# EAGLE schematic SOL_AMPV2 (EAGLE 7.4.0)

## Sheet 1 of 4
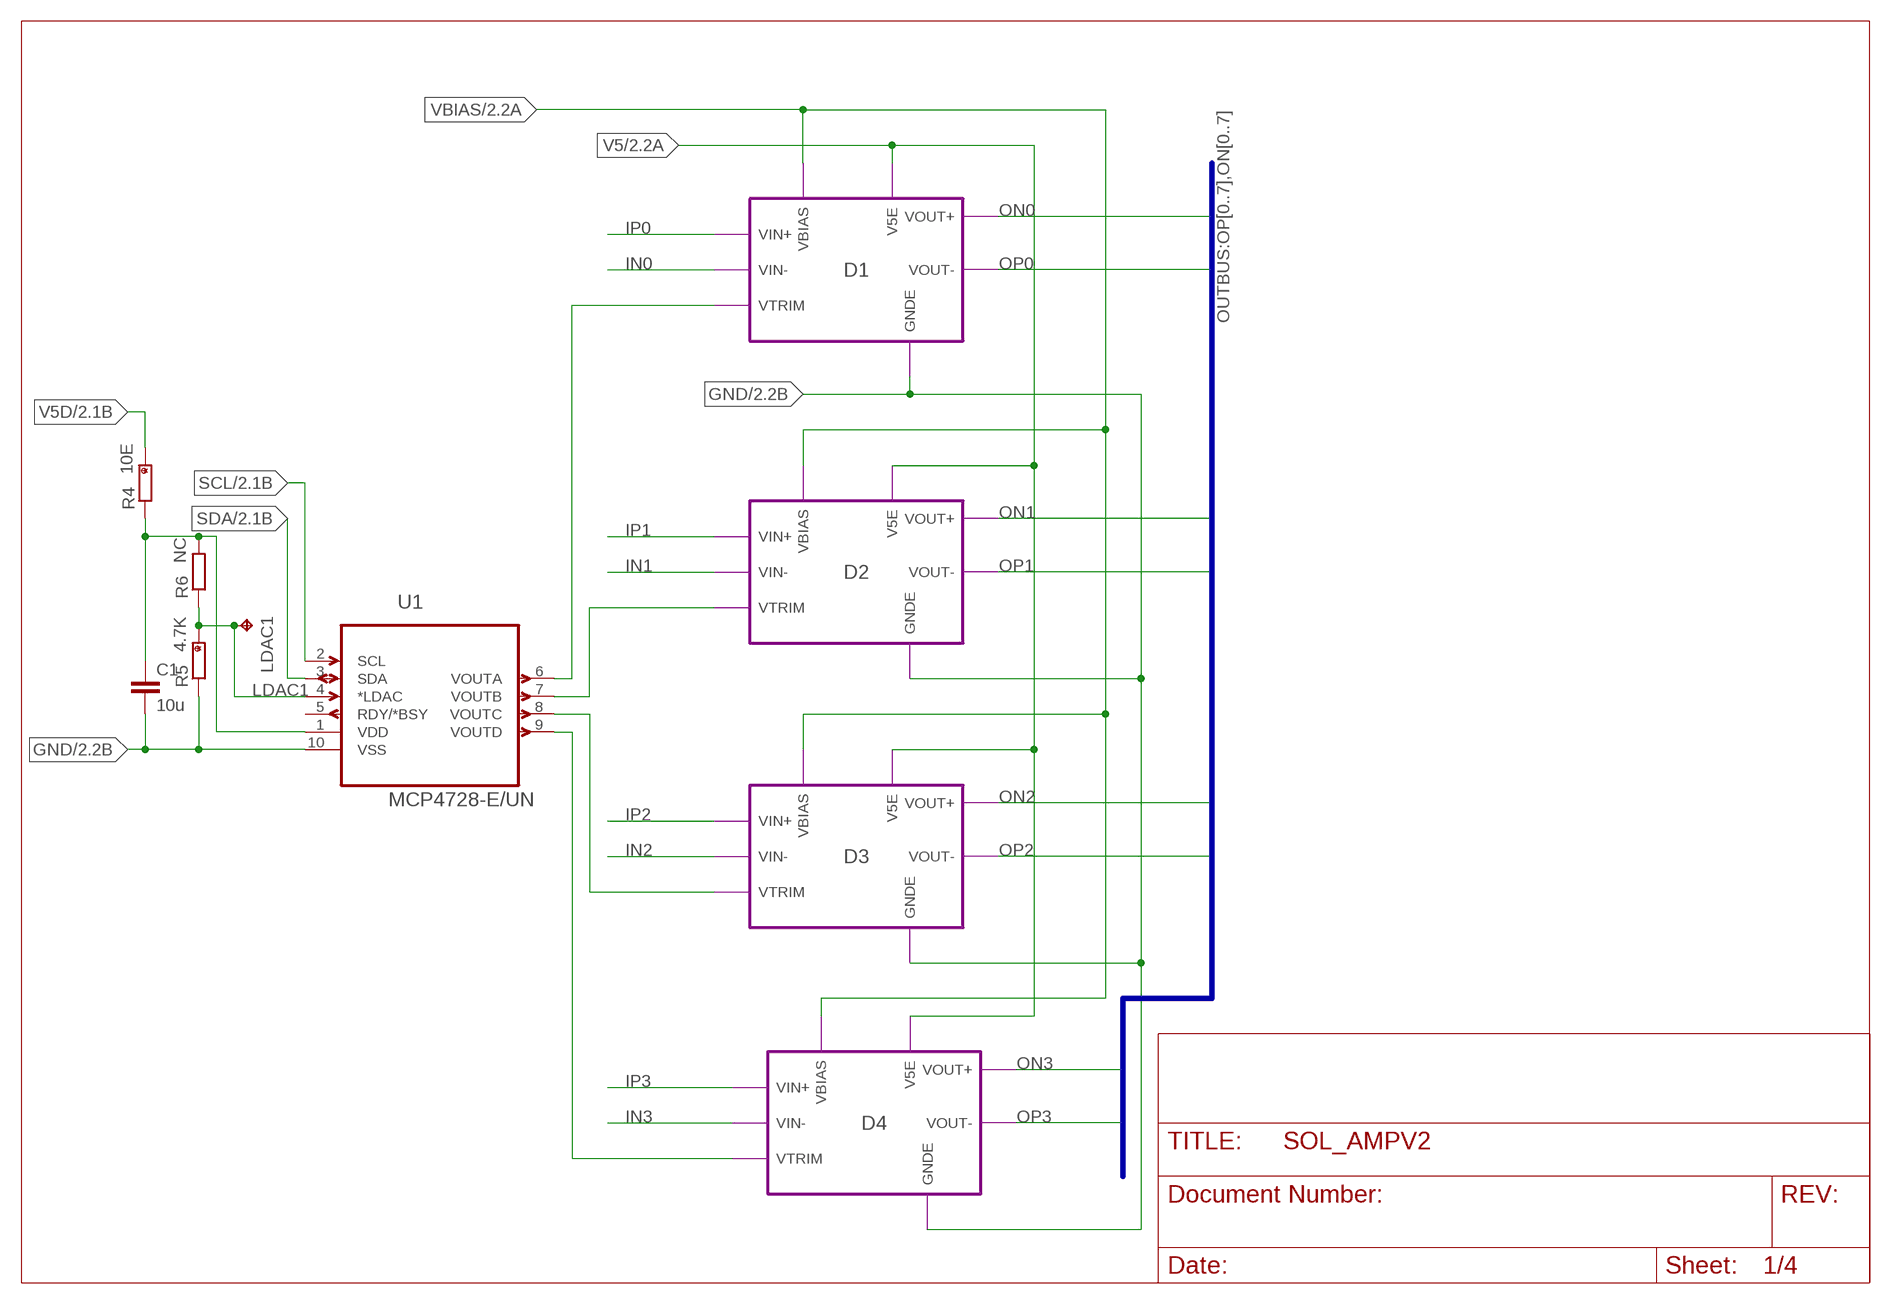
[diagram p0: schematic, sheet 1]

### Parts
C1  10u  C-EUC0805  [C0805]
LDAC1  UA_TPPAD1-13  [UA_P1-13]
R4  10E  R_HAND  [R0805H]
R5  4.7K  R_HAND  [R0805H]
R6  NC  R-EU_R0402  [R0402]
U1  MCP4728-E/UN  [SOP50P490X110-10N]

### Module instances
D2 = DIFFAMP
D1 = DIFFAMP
D3 = DIFFAMP
D4 = DIFFAMP

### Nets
GND: C1.2 R5.1 U1.10(VSS) ; port D2.GNDE D3.GNDE D4.GNDE D1.GNDE ; also sheet 2,3,4
IN0: port D1.VIN- ; also sheet 3
IN1: port D2.VIN- ; also sheet 3
IN2: port D3.VIN- ; also sheet 3
IN3: port D4.VIN- ; also sheet 3
IP0: port D1.VIN+ ; also sheet 3
IP1: port D2.VIN+ ; also sheet 3
IP2: port D3.VIN+ ; also sheet 3
IP3: port D4.VIN+ ; also sheet 3
LDAC1: LDAC1.TP R5.2 R6.1 U1.4(*LDAC)
N$1: C1.1 R4.1 R6.2 U1.1(VDD)
ON0: port D1.VOUT+ ; also sheet 3
ON1: port D2.VOUT+ ; also sheet 3
ON2: port D3.VOUT+ ; also sheet 3
ON3: port D4.VOUT+ ; also sheet 3
OP0: port D1.VOUT- ; also sheet 3
OP1: port D2.VOUT- ; also sheet 3
OP2: port D3.VOUT- ; also sheet 3
OP3: port D4.VOUT- ; also sheet 3
SCL: U1.2(SCL) ; also sheet 2,4
SDA: U1.3(SDA) ; also sheet 2,4
V5: port D2.V5E D3.V5E D4.V5E D1.V5E ; also sheet 2,4
V5D: R4.2 ; also sheet 2,4
VBIAS: port D2.VBIAS D3.VBIAS D4.VBIAS D1.VBIAS ; also sheet 2,4
VTR1: U1.6(VOUTA) ; port D1.VTRIM
VTR2: U1.7(VOUTB) ; port D2.VTRIM
VTR3: U1.8(VOUTC) ; port D3.VTRIM
VTR4: U1.9(VOUTD) ; port D4.VTRIM
Unconnected: U1.5(RDY/*BSY)

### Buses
OUTBUS:OP[0..7],ON[0..7]

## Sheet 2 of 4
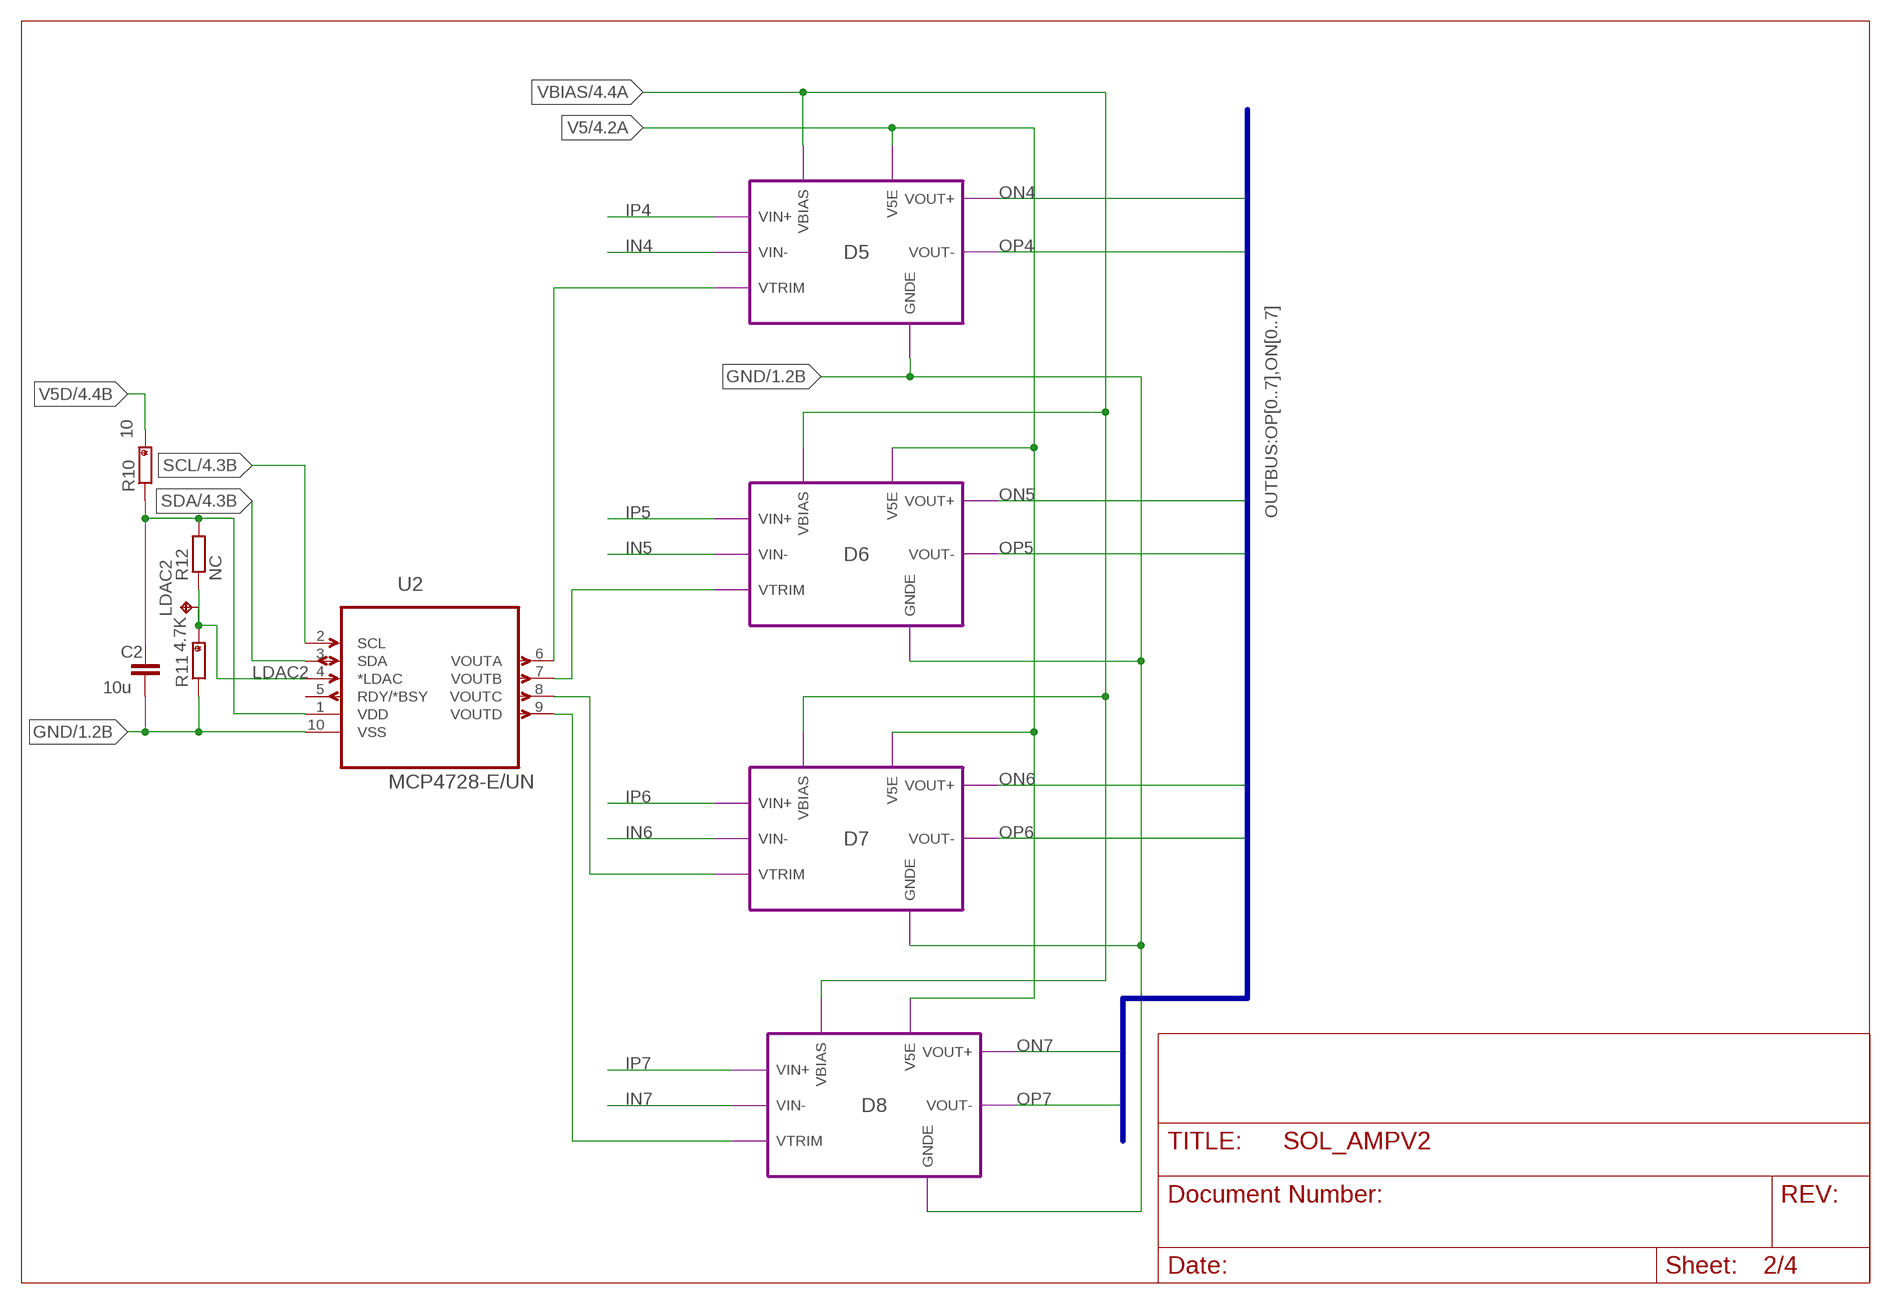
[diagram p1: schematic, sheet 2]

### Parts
C2  10u  C-EUC0805  [C0805]
LDAC2  UA_TPPAD1-13  [UA_P1-13]
R10  10  R_HAND  [R0805H]
R11  4.7K  R_HAND  [R0805H]
R12  NC  R-EU_R0402  [R0402]
U2  MCP4728-E/UN  [SOP50P490X110-10N]

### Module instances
D5 = DIFFAMP
D6 = DIFFAMP
D7 = DIFFAMP
D8 = DIFFAMP

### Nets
GND: C2.2 R11.1 U2.10(VSS) ; port D6.GNDE D7.GNDE D8.GNDE D5.GNDE ; also sheet 1,3,4
IN4: port D5.VIN- ; also sheet 3
IN5: port D6.VIN- ; also sheet 3
IN6: port D7.VIN- ; also sheet 3
IN7: port D8.VIN- ; also sheet 3
IP4: port D5.VIN+ ; also sheet 3
IP5: port D6.VIN+ ; also sheet 3
IP6: port D7.VIN+ ; also sheet 3
IP7: port D8.VIN+ ; also sheet 3
LDAC2: LDAC2.TP R11.2 R12.1 U2.4(*LDAC)
N$11: C2.1 R10.1 R12.2 U2.1(VDD)
ON4: port D5.VOUT+ ; also sheet 3
ON5: port D6.VOUT+ ; also sheet 3
ON6: port D7.VOUT+ ; also sheet 3
ON7: port D8.VOUT+ ; also sheet 3
OP4: port D5.VOUT- ; also sheet 3
OP5: port D6.VOUT- ; also sheet 3
OP6: port D7.VOUT- ; also sheet 3
OP7: port D8.VOUT- ; also sheet 3
SCL: U2.2(SCL) ; also sheet 1,4
SDA: U2.3(SDA) ; also sheet 1,4
V5: port D5.V5E D6.V5E D7.V5E D8.V5E ; also sheet 1,4
V5D: R10.2 ; also sheet 1,4
VBIAS: port D6.VBIAS D7.VBIAS D8.VBIAS D5.VBIAS ; also sheet 1,4
VTR5: U2.6(VOUTA) ; port D5.VTRIM
VTR6: U2.7(VOUTB) ; port D6.VTRIM
VTR7: U2.8(VOUTC) ; port D7.VTRIM
VTR8: U2.9(VOUTD) ; port D8.VTRIM
Unconnected: U2.5(RDY/*BSY)

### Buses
OUTBUS:OP[0..7],ON[0..7]

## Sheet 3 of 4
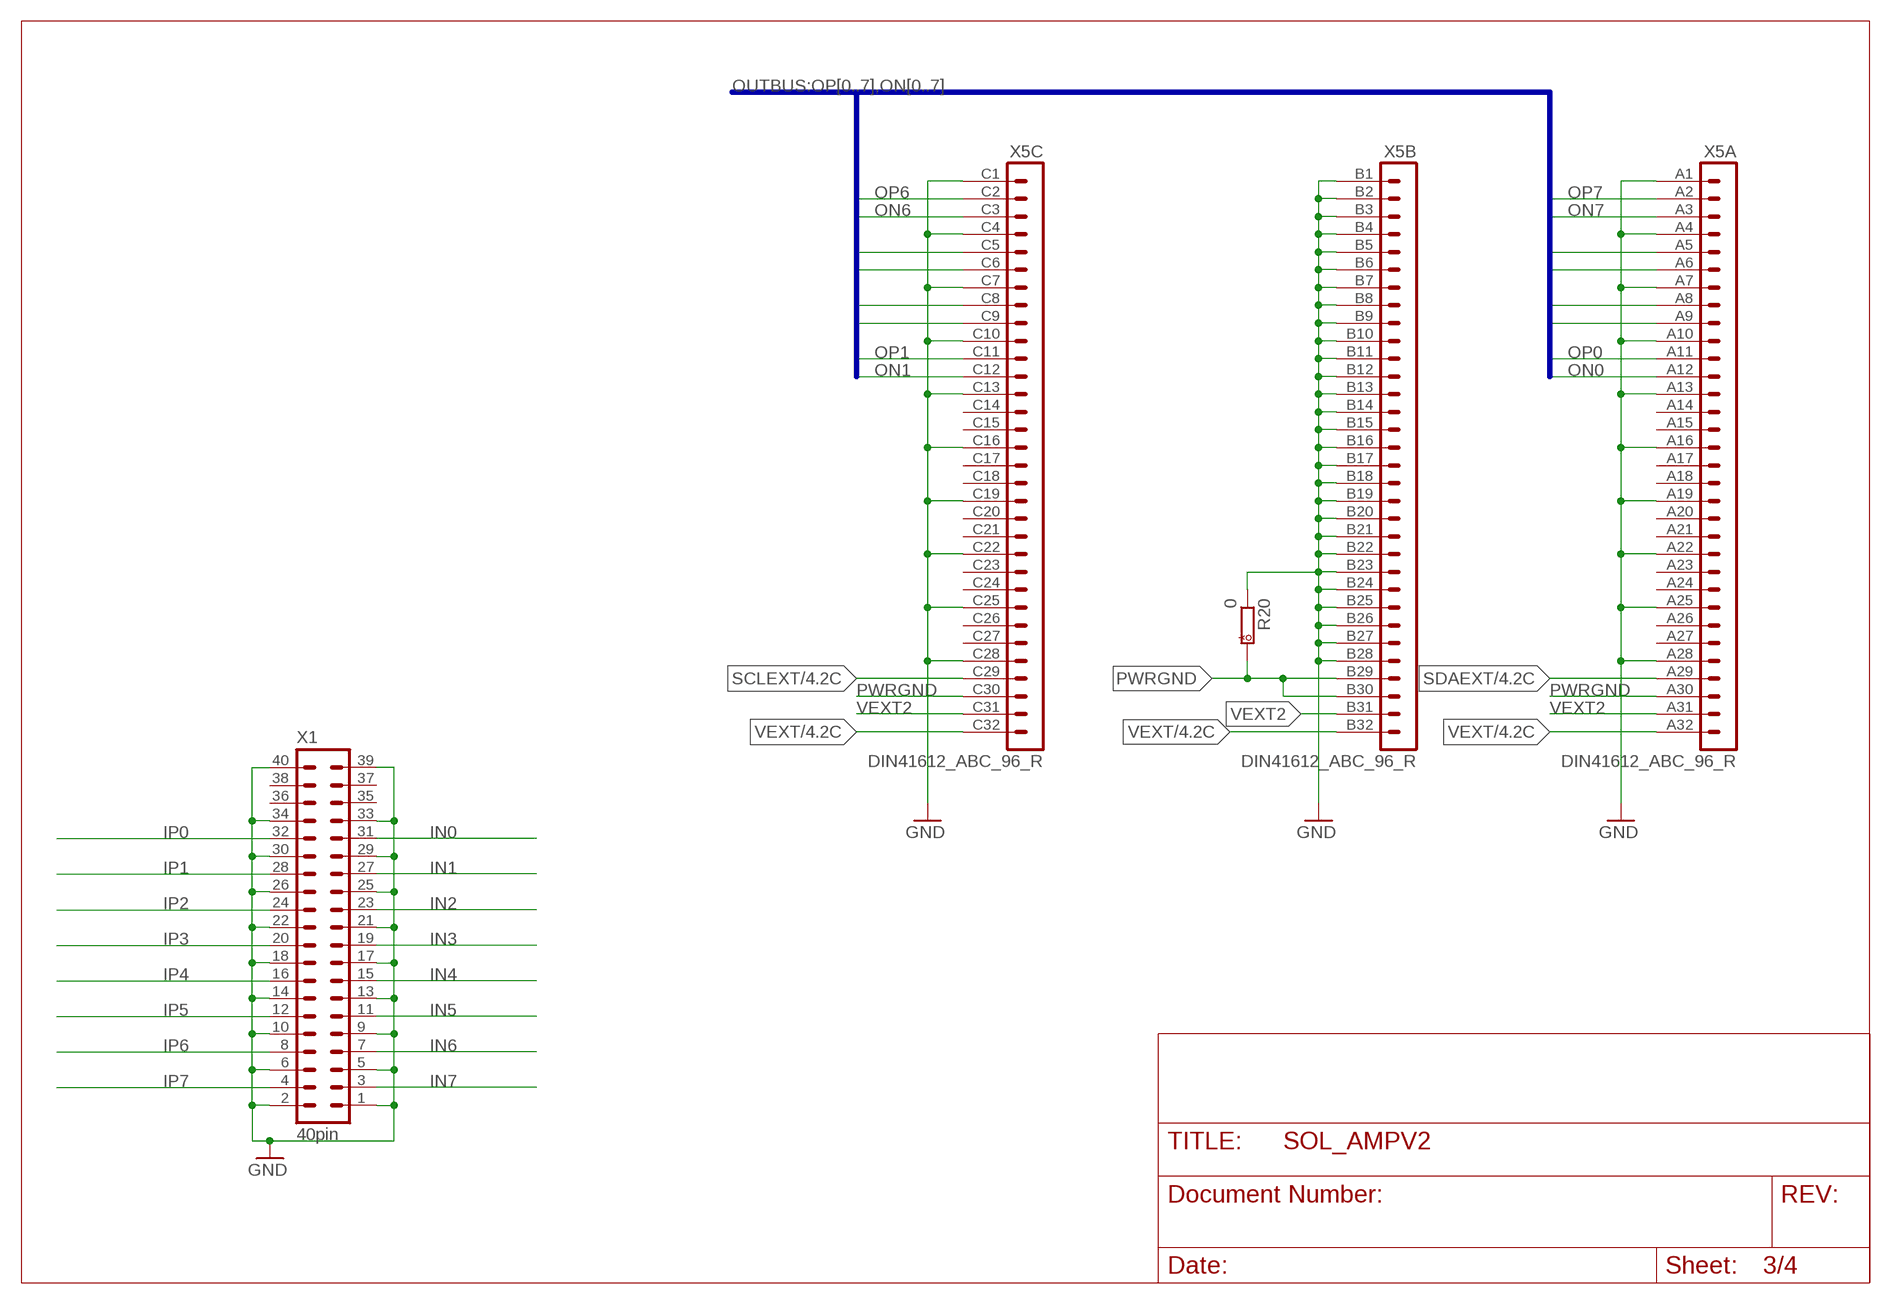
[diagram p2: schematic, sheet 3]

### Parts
R20  0  R_HAND  [R0805H]
X1  40pin  ML40L  [ML40L]
X5  DIN41612_ABC_96_R  [DIN41612_96RC]

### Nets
GND: R20.1 X1.1 X1.2 X1.5 X1.6 X1.9 X1.10 X1.13 X1.14 X1.17 X1.18 X1.21 X1.22 X1.25 X1.26 X1.29 X1.30 X1.33 X1.34 X1.39 X1.40 X5.A1 X5.A4 X5.A7 X5.A10 X5.A13 X5.A16 X5.A19 X5.A22 X5.A25 X5.A28 X5.B1 X5.B2 X5.B3 X5.B4 X5.B5 X5.B6 X5.B7 X5.B8 X5.B9 X5.B10 X5.B11 X5.B12 X5.B13 X5.B14 X5.B15 X5.B16 X5.B17 X5.B18 X5.B19 X5.B20 X5.B21 X5.B22 X5.B23 X5.B24 X5.B25 X5.B26 X5.B27 X5.B28 X5.C1 X5.C4 X5.C7 X5.C10 X5.C13 X5.C16 X5.C19 X5.C22 X5.C25 X5.C28 ; also sheet 1,2,4
IN0: X1.31 ; also sheet 1
IN1: X1.27 ; also sheet 1
IN2: X1.23 ; also sheet 1
IN3: X1.19 ; also sheet 1
IN4: X1.15 ; also sheet 2
IN5: X1.11 ; also sheet 2
IN6: X1.7 ; also sheet 2
IN7: X1.3 ; also sheet 2
IP0: X1.32 ; also sheet 1
IP1: X1.28 ; also sheet 1
IP2: X1.24 ; also sheet 1
IP3: X1.20 ; also sheet 1
IP4: X1.16 ; also sheet 2
IP5: X1.12 ; also sheet 2
IP6: X1.8 ; also sheet 2
IP7: X1.4 ; also sheet 2
ON0: X5.A12 ; also sheet 1
ON1: X5.C12 ; also sheet 1
ON2: X5.A9 ; also sheet 1
ON3: X5.C9 ; also sheet 1
ON4: X5.A6 ; also sheet 2
ON5: X5.C6 ; also sheet 2
ON6: X5.C3 ; also sheet 2
ON7: X5.A3 ; also sheet 2
OP0: X5.A11 ; also sheet 1
OP1: X5.C11 ; also sheet 1
OP2: X5.A8 ; also sheet 1
OP3: X5.C8 ; also sheet 1
OP4: X5.A5 ; also sheet 2
OP5: X5.C5 ; also sheet 2
OP6: X5.C2 ; also sheet 2
OP7: X5.A2 ; also sheet 2
PWRGND: R20.2 X5.A30 X5.B29 X5.B30 X5.C30
SCLEXT: X5.C29 ; also sheet 4
SDAEXT: X5.A29 ; also sheet 4
VEXT: X5.A32 X5.B32 X5.C32 ; also sheet 4
VEXT2: X5.A31 X5.B31 X5.C31
Unconnected: X1.35 X1.36 X1.37 X1.38 X5.A14 X5.A15 X5.A17 X5.A18 X5.A20 X5.A21 X5.A23 X5.A24 X5.A26 X5.A27 X5.C14 X5.C15 X5.C17 X5.C18 X5.C20 X5.C21 X5.C23 X5.C24 X5.C26 X5.C27

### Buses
OUTBUS:OP[0..7],ON[0..7]

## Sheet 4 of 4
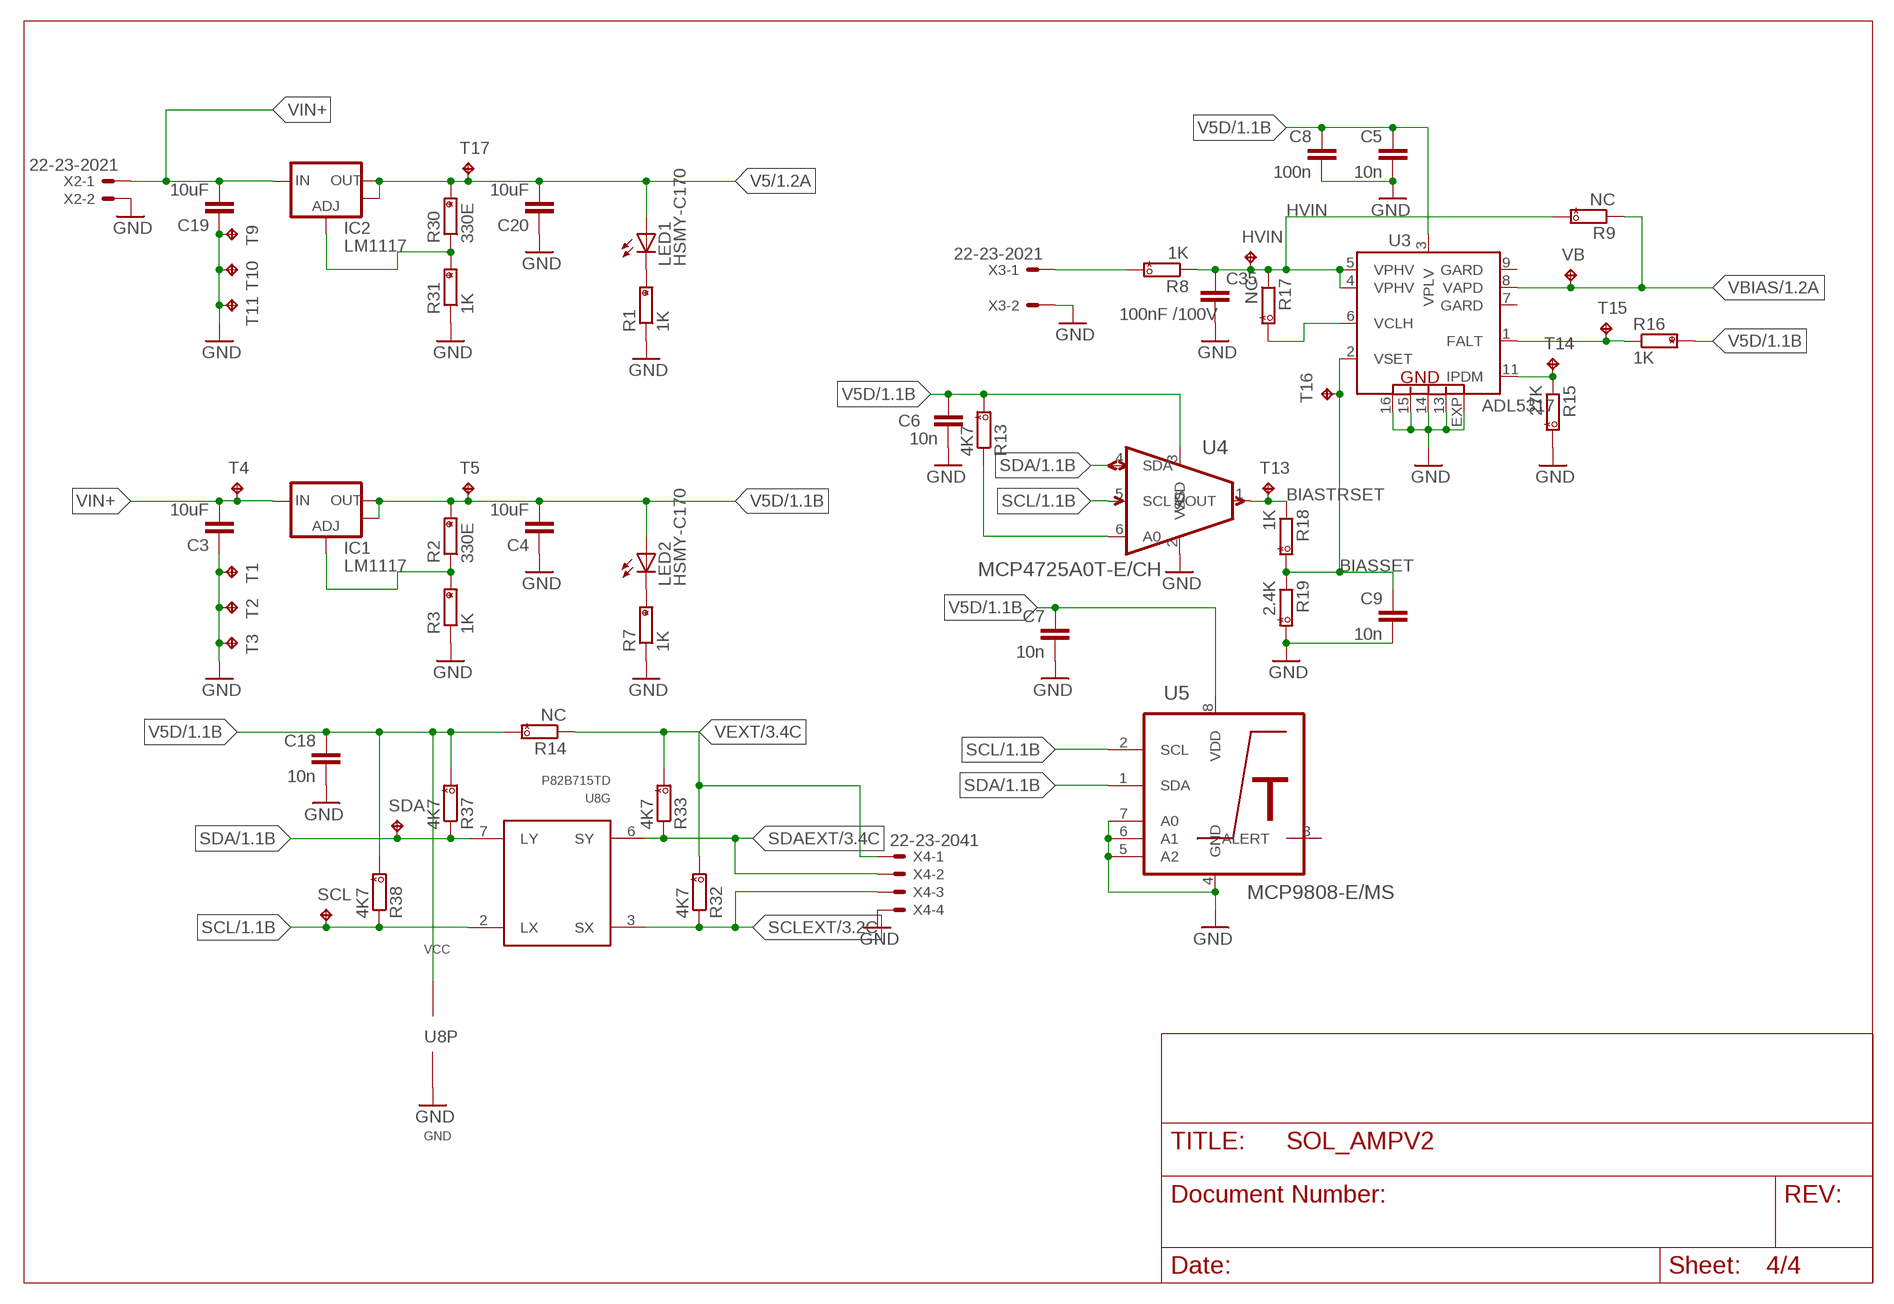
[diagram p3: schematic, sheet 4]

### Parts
C3  10uF  C-EUC0805  [C0805]
C4  10uF  C-EUC0805  [C0805]
C5  10n  C-EUC0805  [C0805]
C6  10n  C-EUC0805  [C0805]
C7  10n  C-EUC0805  [C0805]
C8  100n  C-EUC0805  [C0805]
C9  10n  C-EUC0805  [C0805]
C18  10n  C-EUC0805  [C0805]
C19  10uF  C-EUC0805  [C0805]
C20  10uF  C-EUC0805  [C0805]
C35  100nF /100V  C-EUC0805K  [C0805K]
HVIN  UA_TPPAD1-13  [UA_P1-13]
IC1  LM1117  V_REG_LM1117SOT223  [SOT223]
IC2  LM1117  V_REG_LM1117SOT223  [SOT223]
LED1  HSMY-C170  LEDCHIP-LED0805  [CHIP-LED0805]
LED2  HSMY-C170  LEDCHIP-LED0805  [CHIP-LED0805]
R1  1K  R_HAND  [R0805H]
R2  330E  R_HAND  [R0805H]
R3  1K  R_HAND  [R0805H]
R7  1K  R_HAND  [R0805H]
R8  1K  R_HAND  [R0805H]
R9  NC  R_HAND  [R0805H]
R13  4K7  R_HAND  [R0805H]
R14  NC  R_HAND  [R0805H]
R15  27K  R_HAND  [R0805H]
R16  1K  R_HAND  [R0805H]
R17  NC  R_HAND  [R0805H]
R18  1K  R_HAND  [R0805H]
R19  2.4K  R_HAND  [R0805H]
R30  330E  R_HAND  [R0805H]
R31  1K  R_HAND  [R0805H]
R32  4K7  R_HAND  [R0805H]
R33  4K7  R_HAND  [R0805H]
R37  4K7  R_HAND  [R0805H]
R38  4K7  R_HAND  [R0805H]
SCL  UA_TPPAD1-13  [UA_P1-13]
SDA  UA_TPPAD1-13  [UA_P1-13]
T1  UA_TPPAD1-13  [UA_P1-13]
T2  UA_TPPAD1-13  [UA_P1-13]
T3  UA_TPPAD1-13  [UA_P1-13]
T4  UA_TPPAD1-13  [UA_P1-13]
T5  UA_TPPAD1-13  [UA_P1-13]
T9  UA_TPPAD1-13  [UA_P1-13]
T10  UA_TPPAD1-13  [UA_P1-13]
T11  UA_TPPAD1-13  [UA_P1-13]
T13  UA_TPPAD1-13  [UA_P1-13]
T14  UA_TPPAD1-13  [UA_P1-13]
T15  UA_TPPAD1-13  [UA_P1-13]
T16  UA_TPPAD1-13  [UA_P1-13]
T17  UA_TPPAD1-13  [UA_P1-13]
U3  ADL5317  [LFCSP_LQ-16_MANSOL]
U4  MCP4725A0T-E/CH  [SOT95P270X145-6N]
U5  MCP9808-E/MS  [SOP65P490X110-8N]
U8  P82B715TD  82B715TD  [SO8]
VB  UA_TPPAD1-13  [UA_P1-13]
X2  22-23-2021  [22-23-2021]
X3  22-23-2021  [22-23-2021]
X4  22-23-2041  [22-23-2041]

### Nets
BIASSET: C9.1 R18.2 R19.1 T16.TP U3.2(VSET)
BIASTRSET: R18.1 T13.TP U4.1(VOUT)
GND: C3.1 C4.1 C5.2 C6.2 C7.2 C8.2 C9.2 C18.2 C19.1 C20.1 C35.2 R1.1 R3.1 R7.1 R15.2 R19.2 R31.1 T1.TP T2.TP T3.TP T9.TP T10.TP T11.TP U3.13(GND) U3.14(GND) U3.15(GND) U3.16(GND) U3.EXP(GND) U4.2(VSS) U5.4(GND) U5.5(A2) U5.6(A1) U5.7(A0) U8.4(P:GND) X2.2 X3.2 X4.4 ; also sheet 1,2,3
HVIN: C35.1 HVIN.TP R8.1 R9.2 R17.1 U3.4(VPHV) U3.5(VPHV)
N$2: IC1.1(ADJ) R2.1 R3.2
N$3: LED1.C R1.2
N$4: LED2.C R7.2
N$5: R8.2 X3.1
N$7: R15.1 T14.TP U3.11(IPDM)
N$9: R17.2 U3.6(VCLH)
N$10: R13.1 U4.6(A0)
N$13: R16.1 T15.TP U3.1(FALT)
N$20: IC2.1(ADJ) R30.1 R31.2
SCL: R38.1 SCL.TP U4.5(SCL) U5.2(SCL) U8.2(G:LX) ; also sheet 1,2
SCLEXT: R32.1 U8.3(G:SX) X4.3 ; also sheet 3
SDA: R37.1 SDA.TP U4.4(SDA) U5.1(SDA) U8.7(G:LY) ; also sheet 1,2
SDAEXT: R33.1 U8.6(G:SY) X4.2 ; also sheet 3
V5: C20.2 IC2.2(OUT) IC2.4(OUT) LED1.A R30.2 T17.TP ; also sheet 1,2
V5D: C4.2 C5.1 C6.1 C7.1 C8.1 C18.1 IC1.2(OUT) IC1.4(OUT) LED2.A R2.2 R13.2 R14.2 R16.2 R37.2 R38.2 T5.TP U3.3(VPLV) U4.3(VDD) U5.8(VDD) U8.8(P:VCC) ; also sheet 1,2
VBIAS: R9.1 U3.8(VAPD) VB.TP ; also sheet 1,2
VEXT: R14.1 R32.2 R33.2 X4.1 ; also sheet 3
VIN+: C3.2 C19.2 IC1.3(IN) IC2.3(IN) T4.TP X2.1
Unconnected: U3.7(GARD) U3.9(GARD) U5.3(ALERT) U8.1(NC:NC) U8.5(NC:NC)

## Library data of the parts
C1 C2 C35 = rcl:C-EU: CAPACITOR, European symbol
C3-C9 C18-C20 = rcl:C-EU: CAPACITOR, European symbol; PARTNO: *
HVIN LDAC1 LDAC2 SCL SDA T1-T5 T9-T11 T13-T17 VB = UA_v2:UA_TP: Test pad; PARTNO: *
IC1 IC2 = SparkFunEagle-6-6-07:V_REG_LM1117: Voltage Regulator LM1117 Standard adjustable voltage regulator but in SMD form. Spark Fun Electronics SKU : COM-00595
LED1 LED2 = led:LED: LED
R1-R3 R7-R9 R13-R20 R30-R33 R37 R38 = UA_v2:R_HAND; PARTNO: *
R4 R5 R10 R11 = UA_v2:R_HAND
R6 R12 = resistor:R-EU_: RESISTOR, European symbol
U1 U2 = MCP4728:MCP4728-E/UN: IC, DAC, 12BIT, QUAD; MPN: MCP4728-E/UN; OC_FARNELL: 1800217; OC_NEWARK: 08R1808; PACKAGE: MSOP-10; SUPPLIER: MICROCHIP
U3 = adl783:ADL5317: APD voltage regulator; OC_FARNELL: 2462433
U4 = MCP4725A0T:MCP4725A0T-E/CH: 12-Bit Digital-to-Analog Converter with EEPROM; MPN: MCP4725A0T-E/CH; OC_FARNELL: 1578449; OC_NEWARK: 77M3032; PACKAGE: SOT-23-6; SUPPLIER: Microchip
U5 = MCP4725A0T:MCP9808-E/MS: Digital Temperature Sensor,MSOP-8; MPN: MCP9808-E/MS; OC_FARNELL: 2080523; OC_NEWARK: 89T8871; PACKAGE: MSOP-8; SUPPLIER: MICROCHIP
U8 = UA_v2:82B715: I2C bus extender; PARTNO: P82B715TD,112
X1 = con-harting-ml:ML40: HARTING; OC_FARNELL: unknown; OC_NEWARK: unknown
X2 X3 = con-molex:22-23-2021: .100" (2.54mm) Center Header - 2 Pin; MF: MOLEX; MPN: 22-23-2021; OC_FARNELL: 1462926; OC_NEWARK: 25C3832
X4 = con-molex:22-23-2041: .100" (2.54mm) Center Header - 4 Pin; MF: MOLEX; MPN: 22-23-2041; OC_FARNELL: 1462920; OC_NEWARK: 38C0355
X5 = con3:DIN41612_ABC_96_R

## Module DIFFAMP
Ports: VIN+(in) VIN-(in) VTRIM(in) V5E(pwr) GNDE(pwr) VBIAS(in) VOUT+(out) VOUT-(out)
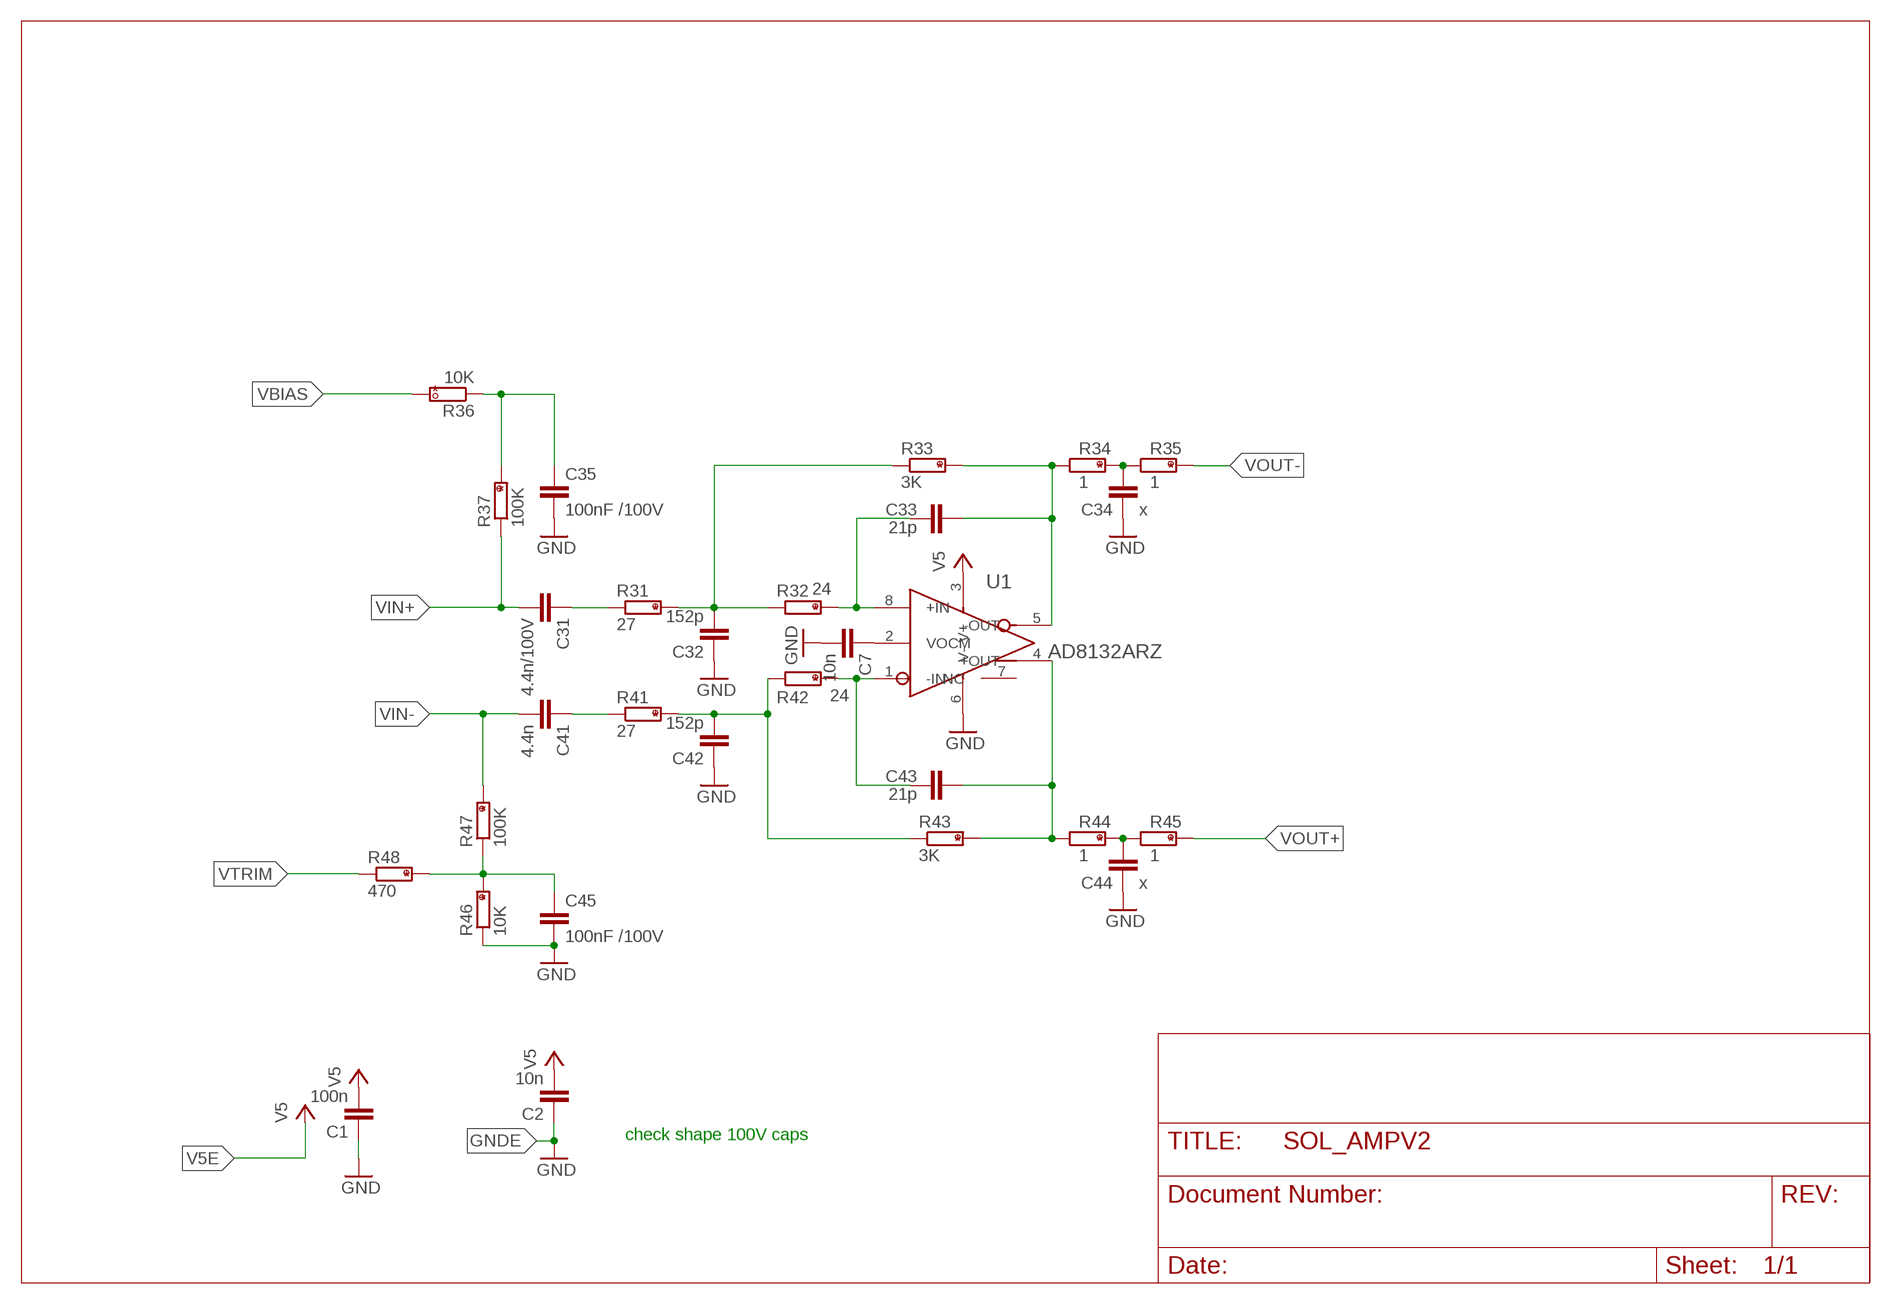
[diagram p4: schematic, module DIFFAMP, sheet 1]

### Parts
C1  100n  C-EUC0805K  [C0805K]
C2  10n  C-EUC0805K  [C0805K]
C7  10n  C-EUC0805K  [C0805K]
C31  4.4n/100V  C-EUC0805K  [C0805K]
C32  152p  C-EUC0805K  [C0805K]
C33  21p  C-EUC0805K  [C0805K]
C34  x  C-EUC0805K  [C0805K]
C35  100nF /100V  C-EUC0805K  [C0805K]
C41  4.4n  C-EUC0805K  [C0805K]
C42  152p  C-EUC0805K  [C0805K]
C43  21p  C-EUC0805K  [C0805K]
C44  x  C-EUC0805K  [C0805K]
C45  100nF /100V  C-EUC0805K  [C0805K]
R31  27  R_HAND  [R0805H]
R32  24  R_HAND  [R0805H]
R33  3K  R_HAND  [R0805H]
R34  1  R_HAND  [R0805H]
R35  1  R_HAND  [R0805H]
R36  10K  R_HAND  [R0805H]
R37  100K  R_HAND  [R0805H]
R41  27  R_HAND  [R0805H]
R42  24  R_HAND  [R0805H]
R43  3K  R_HAND  [R0805H]
R44  1  R_HAND  [R0805H]
R45  1  R_HAND  [R0805H]
R46  10K  R_HAND  [R0805H]
R47  100K  R_HAND  [R0805H]
R48  470  R_HAND  [R0805H]
U1  AD8132ARZ  [SOIC127P600X175-8N]

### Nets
AOUT+: C43.2 R43.2 R44.1 U1.4(+OUT)
AOUT-: C33.2 R33.2 R34.1 U1.5(-OUT)
FB+: C32.2 R31.2 R32.1 R33.1
FB-: C42.2 R41.2 R42.1 R43.1
GNDE: C1.1 C2.1 C7.2 C32.1 C34.1 C35.2 C42.1 C44.1 C45.2 R46.1 U1.6(V-) ; supply symbol labelled GND
N$1: C34.2 R34.2 R35.1
N$2: C7.1 U1.2(VOCM)
N$3: C44.2 R44.2 R45.1
N$4: C43.1 R42.2 U1.1(-IN)
N$5: C33.1 R32.2 U1.8(+IN)
N$10: C41.1 R41.1
R31: C31.1 R31.1
V5E: C1.2 C2.2 U1.3(V+) ; supply symbol labelled V5
VB+: C35.1 R36.1 R37.2
VB-: C45.1 R46.2 R47.1 R48.2
VBIAS: R36.2
VIN+: C31.2 R37.1
VIN-: C41.2 R47.2
VOUT+: R45.2
VOUT-: R35.2
VTRIM: R48.1
Unconnected: U1.7(NC)

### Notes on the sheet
- check shape 100V caps

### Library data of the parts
C1 C2 C7 C31-C35 C41-C45 = rcl:C-EU: CAPACITOR, European symbol
R31-R37 R41-R48 = UA_v2:R_HAND
U1 = ua_cmp:AD8132ARZ: Low Cost, High Speed Differential Amplifier; MPN: AD8132ARZ; OC_FARNELL: 9426043; OC_NEWARK: 19M8885; PACKAGE: SOIC-8; SUPPLIER: Analog Devices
